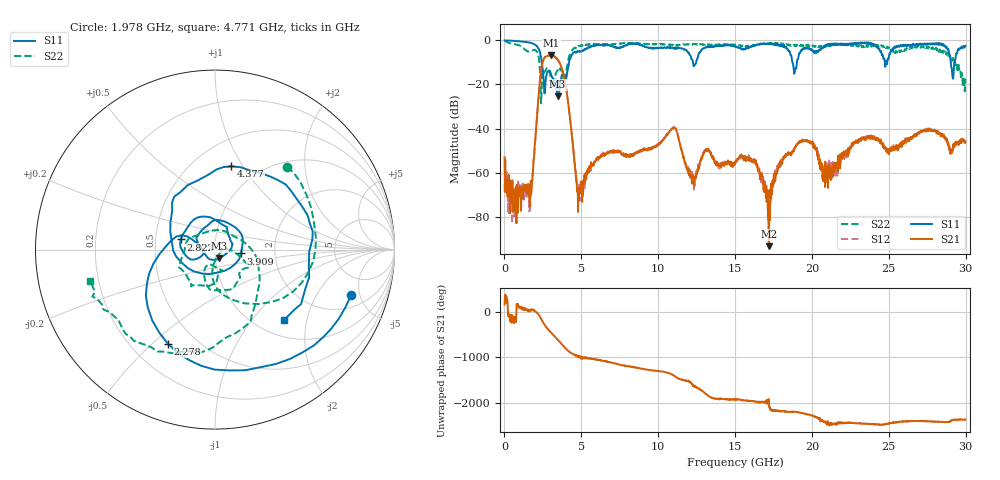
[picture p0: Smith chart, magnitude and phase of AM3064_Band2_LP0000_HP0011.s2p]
# Hz S DB R 50.0
!freq dBS11 angS11 dBS21 angS21 dBS12 angS12 dBS22 angS22
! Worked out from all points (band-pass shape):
!   1600 points, 10 MHz to 29.98 GHz, reference 50 ohm
!   highest |S21| = -6.77 dB at 3.046 GHz (marker M1); lowest = -93.3 dB at 17.2 GHz (marker M2)
!   |S21| within 3 dB of the highest: 2.486 GHz to 3.552 GHz (1.066 GHz wide, 35.3 % of centre)
!   lowest |S11| = -25.3 dB at 3.459 GHz (marker M3), VSWR 1.11, Z = 52.2 - j5.09 ohm
!   |S11| at or under -10 dB: 2.425 GHz to 4.206 GHz (1.781 GHz wide, 53.7 % of centre); 18.73 GHz to 19.02 GHz (288 MHz wide, 1.53 % of centre); 29.03 GHz to 29.26 GHz (229.4 MHz wide, 0.787 % of centre)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
!   |S22| runs from -28.5 to -0.2 dB; largest |S21 - S12| = 0.017
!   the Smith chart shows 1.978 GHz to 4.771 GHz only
!   S11 on the Smith chart (normalised r, x): 1.978 GHz: 2.96, -4.15; 2.278 GHz: 0.35, -0.56; 2.822 GHz: 0.68, +0.08; 3.909 GHz: 1.34, -0.06; 4.377 GHz: 0.75, +0.89; 4.771 GHz: 1.32, -1.48
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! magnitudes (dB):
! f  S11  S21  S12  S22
! 10 MHz  0.0  -53.0  -65.2  -0.2
! 1.622 GHz  -0.9  -72.9  -77.0  -5.1
! 1.978 GHz  -1.9  -47.3  -47.7  -4.2
! 2.278 GHz  -4.6  -20.4  -20.4  -10.6
! 2.822 GHz  -14.0  -7.0  -6.9  -12.8
! 3.046 GHz  -15.7  -6.8  -6.8  -18.9
! 3.459 GHz  -25.3  -8.7  -8.6  -13.5
! 3.909 GHz  -16.7  -17.8  -17.8  -19.2
! 4.377 GHz  -6.5  -42.8  -42.7  -4.7
! 4.771 GHz  -5.2  -68.8  -67.9  -2.9
! 5.015 GHz  -4.9  -67.3  -67.3  -2.5
! 6.308 GHz  -2.1  -52.1  -52.7  -1.7
! 10 GHz  -3.4  -47.3  -47.3  -1.7
! 11.09 GHz  -4.0  -39.7  -39.6  -1.9
! 12.31 GHz  -11.7  -63.8  -62.1  -1.6
! 15 GHz  -2.6  -55.6  -55.1  -1.9
! 17.2 GHz  -1.6  -93.3  -80.7  -1.6
! 18.23 GHz  -3.1  -52.7  -52.2  -1.7
! 19.99 GHz  -4.2  -46.7  -47.2  -2.1
! 20.89 GHz  -2.1  -61.2  -56.8  -2.9
! 25 GHz  -7.9  -50.8  -50.0  -3.1
! 29.98 GHz  -2.4  -46.0  -47.2  -17.3
